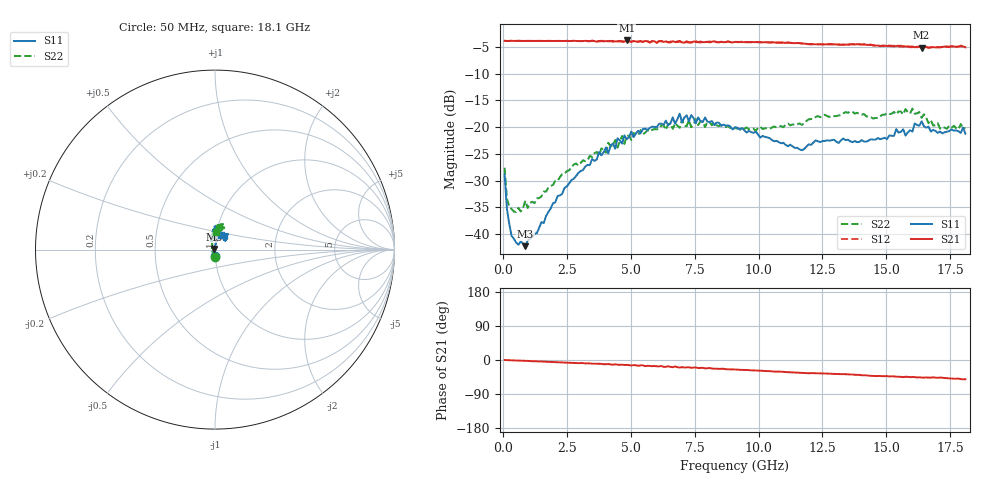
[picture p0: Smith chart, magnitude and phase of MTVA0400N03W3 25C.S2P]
! Network Analyzer HP8720D.06.14 Serial No. US36140669
!  7 Jul 2005  13:24:16
! Frequency  S11  S21  S12  S22
# HZ  S  DB R 50
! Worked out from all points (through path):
!   201 points, 50 MHz to 18.1 GHz, reference 50 ohm
!   highest |S21| = -3.82 dB at 4.833 GHz (marker M1); lowest = -5.2 dB at 16.39 GHz (marker M2)
!   group delay of S21, straight-line fit = 7.89 ps
!   lowest |S11| = -42.2 dB at 862.2 MHz (marker M3), VSWR 1.02, Z = 49.3 + j0.395 ohm
!   |S11| at or under -10 dB: start of sweep to end of sweep
!   |S22| runs from -35.9 to -16.5 dB; largest |S21 - S12| = 0.023
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5e7  -28.81 -94.1  -3.88 -0.0  -3.89 0.1  -27.60 -86.6
1.4025e8  -35.26 -110.4  -3.93 -0.3  -3.92 -0.3  -33.37 -130.1
3.2075e8  -40.29 -140.5  -3.88 -0.7  -3.90 -0.7  -35.30 -159.1
6.8175e8  -41.36 171.6  -3.91 -1.8  -3.92 -1.8  -35.76 173.3
8.6225e8  -42.24 148.8  -3.91 -2.2  -3.92 -2.3  -33.75 166.7
1.22325e9  -39.94 128.8  -3.92 -3.2  -3.92 -3.3  -34.23 147.3
3.1185e9  -28.04 84.1  -3.94 -8.2  -3.96 -8.6  -26.20 114.1
4.382e9  -24.04 79.2  -4.01 -11.3  -3.96 -12.4  -22.42 104.0
4.47225e9  -22.09 75.9  -4.00 -12.4  -3.94 -11.6  -23.84 106.5
4.83325e9  -22.30 84.8  -3.82 -12.9  -3.93 -13.8  -21.68 93.9
6.09675e9  -19.40 81.5  -3.99 -16.8  -3.91 -16.8  -20.30 91.5
6.7285e9  -19.38 88.2  -4.10 -17.2  -4.25 -18.1  -19.25 85.5
6.909e9  -17.49 87.3  -3.90 -19.8  -4.03 -18.9  -20.14 84.2
7.54075e9  -19.29 83.8  -4.11 -19.5  -3.96 -21.3  -18.49 90.2
9.075e9  -20.01 96.4  -4.10 -25.0  -4.09 -25.1  -20.20 81.8
1.169225e10  -24.33 86.8  -4.41 -34.3  -4.40 -34.2  -19.58 81.7
1.21435e10  -22.88 83.1  -4.54 -34.5  -4.50 -34.7  -18.46 81.9
1.512175e10  -21.56 43.6  -4.87 -43.3  -4.73 -43.0  -17.56 82.8
1.602425e10  -20.85 53.5  -4.95 -44.7  -5.07 -46.6  -16.54 72.6
1.638525e10  -18.91 49.9  -5.19 -46.2  -5.04 -45.7  -18.27 70.2
1.674625e10  -20.85 52.7  -5.09 -46.5  -5.18 -47.2  -18.69 71.1
1.81e10  -21.24 66.8  -5.09 -50.7  -5.18 -51.7  -20.19 85.7
